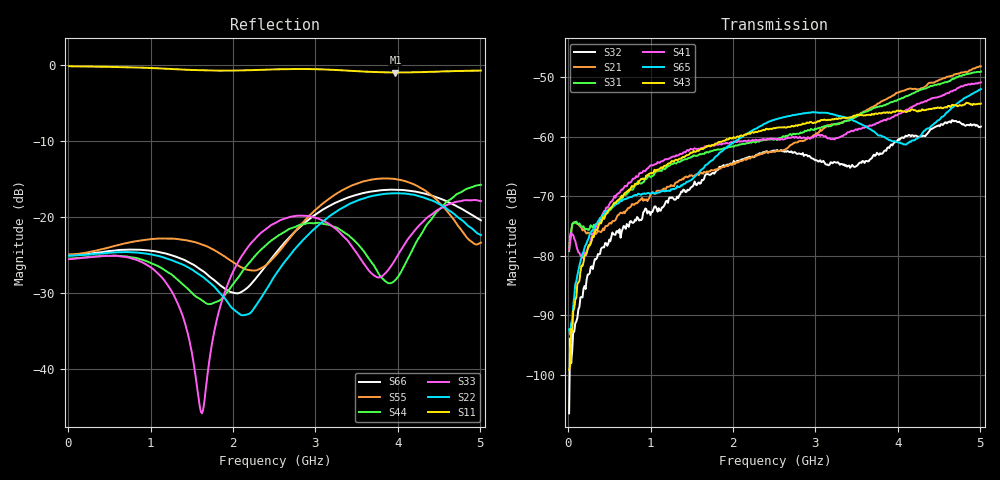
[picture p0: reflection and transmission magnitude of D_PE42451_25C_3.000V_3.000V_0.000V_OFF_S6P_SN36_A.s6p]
! Device ID: PE42451
! Serial: 36
! Insertion: A
! Temp: 25C
! VDD: 3.000
! Control_Hi: 100.000
! Control_Lo: 0.000
! Logic State: OFF
! Port 1: RFC
! Port 2: RF1
! Port 3: RF2
! Port 4: RF3
! Port 5: RF4
! Port 6: RF5
! V1 = 0.00
! V2 = 3.00
! V3 = 3.00
! V4 = 0.00
! IDD: 1.317440e-05
#  Hz  S  RI  R  50
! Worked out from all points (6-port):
!   401 points, 10 MHz to 5.01 GHz, reference 50 ohm
!   strongest paths, dB at 10 MHz, 1.26 GHz, 2.51 GHz, 3.76 GHz, 5.01 GHz:
!     S43: -99.2, -64.1, -58.6, -56.1, -54.4
!     S65: -92.4, -68.8, -57.1, -59.7, -51.9
!     S41: -79.0, -63.4, -60.3, -57.7, -50.8
!     S31: -79.2, -64.6, -60.4, -54.9, -49.0
!     S21: -78.6, -68.2, -62.5, -54.4, -48.1
!     S32: -106.5, -70.2, -62.3, -62.8, -58.3
!   lowest |S11| = -0.9 dB at 3.973 GHz (marker M1), VSWR 18.33, Z = 2.96 - j14.7 ohm
!   |S11| at or under -10 dB: nowhere
